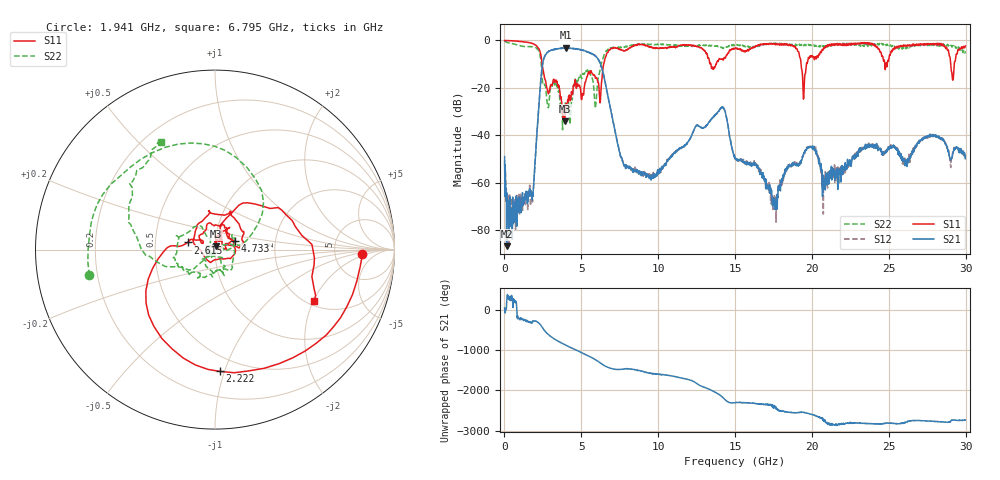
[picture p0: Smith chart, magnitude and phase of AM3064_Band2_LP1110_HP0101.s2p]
# Hz S DB R 50.0
!freq dBS11 angS11 dBS21 angS21 dBS12 angS12 dBS22 angS22
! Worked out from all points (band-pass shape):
!   1600 points, 10 MHz to 29.98 GHz, reference 50 ohm
!   highest |S21| = -3.12 dB at 4.002 GHz (marker M1); lowest = -86.7 dB at 141.2 MHz (marker M2)
!   |S21| within 3 dB of the highest: 2.666 GHz to 5.827 GHz (3.161 GHz wide, 74.4 % of centre)
!   lowest |S11| = -34.1 dB at 3.909 GHz (marker M3), VSWR 1.04, Z = 50.6 + j1.91 ohm
!   |S11| at or under -10 dB: 2.45 GHz to 6.456 GHz (4.006 GHz wide, 90 % of centre); 13.43 GHz to 13.77 GHz (345.4 MHz wide, 2.54 % of centre); 19.29 GHz to 19.64 GHz (349.8 MHz wide, 1.8 % of centre)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
!   |S22| runs from -37.7 to -0.3 dB; largest |S21 - S12| = 0.022
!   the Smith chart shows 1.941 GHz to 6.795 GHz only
!   S11 on the Smith chart (normalised r, x): 1.941 GHz: 10, -2; 2.222 GHz: 0.38, -0.96; 2.615 GHz: 0.73, +0.06; 4.733 GHz: 1.25, +0.12; 6.795 GHz: 2.16, -2.02
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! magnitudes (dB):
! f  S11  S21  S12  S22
! 10 MHz  0.0  -49.0  -50.7  -0.3
! 141.2 MHz  0.0  -86.7  -63.7  -0.7
! 572.3 MHz  -0.2  -70.6  -77.1  -1.5
! 1.941 GHz  -1.7  -56.7  -56.2  -2.9
! 2.222 GHz  -3.4  -29.1  -29.1  -4.3
! 2.615 GHz  -16.0  -6.7  -6.7  -18.9
! 3.909 GHz  -34.1  -3.4  -3.2  -29.5
! 4.002 GHz  -26.7  -3.1  -3.3  -27.0
! 4.733 GHz  -18.2  -3.6  -3.6  -16.6
! 5.015 GHz  -24.9  -4.0  -4.0  -16.1
! 5.933 GHz  -15.9  -6.7  -6.7  -27.7
! 6.795 GHz  -4.1  -25.6  -25.6  -3.5
! 7.826 GHz  -4.4  -52.7  -52.6  -2.8
! 10 GHz  -3.4  -54.4  -55.6  -1.8
! 14.12 GHz  -7.8  -28.1  -28.3  -3.0
! 15 GHz  -3.2  -49.9  -49.9  -2.0
! 17.59 GHz  -1.3  -68.0  -69.7  -1.1
! 19.47 GHz  -24.1  -47.4  -47.9  -2.2
! 19.99 GHz  -6.4  -44.9  -44.9  -1.8
! 20.83 GHz  -3.3  -59.5  -61.9  -2.2
! 25 GHz  -8.0  -45.9  -45.0  -1.6
! 29.98 GHz  -2.3  -49.9  -49.4  -4.6
